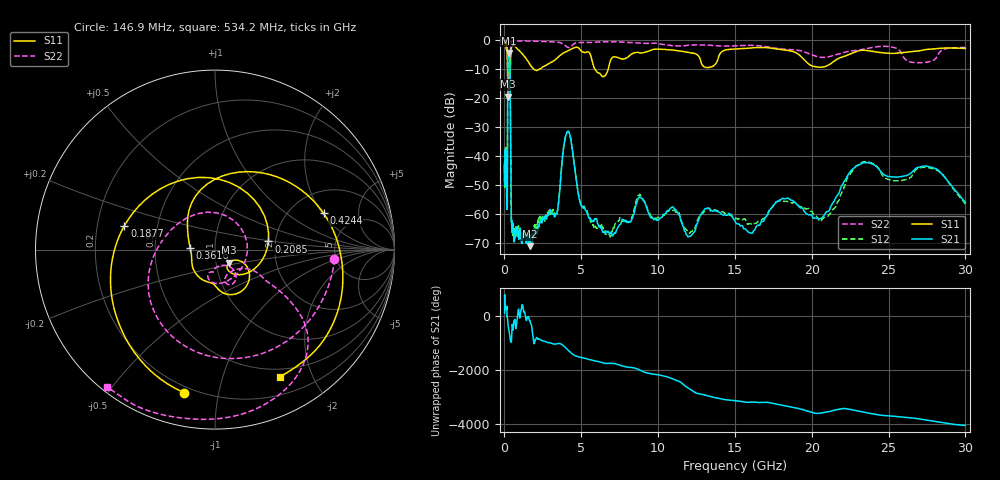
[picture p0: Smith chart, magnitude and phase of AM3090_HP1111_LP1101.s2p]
! Date/Time: Thu, Feb 28, 2019 2:10 PM
! Network Analyzer: Agilent Technologies E8364B Rev: A.07.50.67
! Sweep from 0.010 to 30.000 GHz, 1601 Points, Sweep Type: LOG
! Power Supply: 5.023 V, 0.002 A
# Hz S DB R 50
!freq MagS11 AngS11 MagS21 AngS21 MagS12 AngS12 MagS22 AngS22
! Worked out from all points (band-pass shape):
!   1601 points, 10 MHz to 30 GHz, reference 50 ohm
!   highest |S21| = -4.46 dB at 267.8 MHz (marker M1); lowest = -71.2 dB at 1.63 GHz (marker M2)
!   |S21| within 3 dB of the highest: 220.9 MHz to 350.9 MHz (130 MHz wide, 45.5 % of centre)
!   lowest |S11| = -19.5 dB at 246 MHz (marker M3), VSWR 1.24, Z = 57.6 - j8.52 ohm
!   |S11| at or under -10 dB: 207.1 MHz to 383.9 MHz (176.8 MHz wide, 59.8 % of centre); 1.898 GHz to 2.272 GHz (374.3 MHz wide, 17.9 % of centre); 5.884 GHz to 6.754 GHz (870.1 MHz wide, 13.8 % of centre)
!   |S22| runs from -20.5 to -0.1 dB; largest |S21 - S12| = 0.014
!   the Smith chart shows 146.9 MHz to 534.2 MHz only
!   S11 on the Smith chart (normalised r, x): 146.9 MHz: 0.17, -0.79; 187.7 MHz: 0.32, +0.12; 208.5 MHz: 1.84, +0.18; 361.6 MHz: 0.76, +0.01; 424.4 MHz: 3.01, +2.06; 534.2 MHz: 0.40, -1.55
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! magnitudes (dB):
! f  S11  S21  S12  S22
! 10 MHz  -0.3  -43.6  -45.2  -0.7
! 38.04 MHz  -0.3  -41.0  -40.5  -1.3
! 105.6 MHz  -1.0  -39.7  -39.7  -3.0
! 144.7 MHz  -1.7  -56.5  -57.0  -3.5
! 146.9 MHz  -1.8  -56.4  -57.1  -3.5
! 187.7 MHz  -5.6  -52.6  -49.5  -6.8
! 208.5 MHz  -10.4  -14.4  -14.3  -14.9
! 246 MHz  -19.5  -4.9  -4.8  -18.2
! 267.8 MHz  -14.8  -4.5  -4.4  -19.9
! 361.6 MHz  -17.2  -9.7  -9.7  -7.9
! 424.4 MHz  -3.9  -51.4  -51.8  -0.6
! 534.2 MHz  -2.0  -65.3  -67.0  -0.2
! 550.5 MHz  -1.9  -63.8  -66.2  -0.2
! 1.63 GHz  -8.1  -71.2  -68.9  -0.3
! 2.084 GHz  -10.5  -66.6  -65.2  -0.4
! 3.385 GHz  -6.4  -60.0  -60.3  -0.7
! 4.115 GHz  -3.7  -31.6  -31.5  -2.5
! 5.783 GHz  -8.7  -62.6  -63.7  -0.7
! 7.926 GHz  -6.2  -62.5  -62.7  -0.8
! 16.13 GHz  -2.7  -66.7  -63.8  -1.8
! 23.48 GHz  -3.5  -42.3  -42.1  -3.0
! 30 GHz  -2.9  -56.0  -56.6  -2.5
